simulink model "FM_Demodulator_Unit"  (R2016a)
settings: Solver=ode3  StartTime=0.0  StopTime=6  FixedStep=1/5000000  RelTol=1e-3
libraries: dsparch4 x1

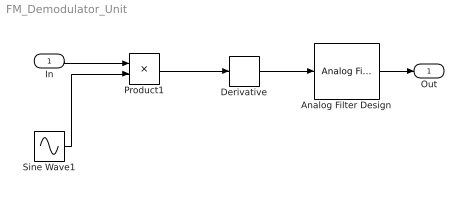
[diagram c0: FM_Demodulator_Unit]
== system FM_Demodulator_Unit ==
  In : Inport
  Analog Filter Design : dsparch4/Analog Filter Design  method=Butterworth  filttype=Lowpass  N=10  Wlo=45000*2*pi  Whi=80  Rp=2  Rs=40
  Derivative : Derivative
  Product1 : Product
  Sine Wave1 : Sin  Frequency=500000*2*pi  Phase=-1.5*pi
  Out : Outport
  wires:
  Product1/1 -> Derivative/1
  Derivative/1 -> Analog Filter Design/1
  Analog Filter Design/1 -> Out/1
  Sine Wave1/1 -> Product1/2
  In/1 -> Product1/1
